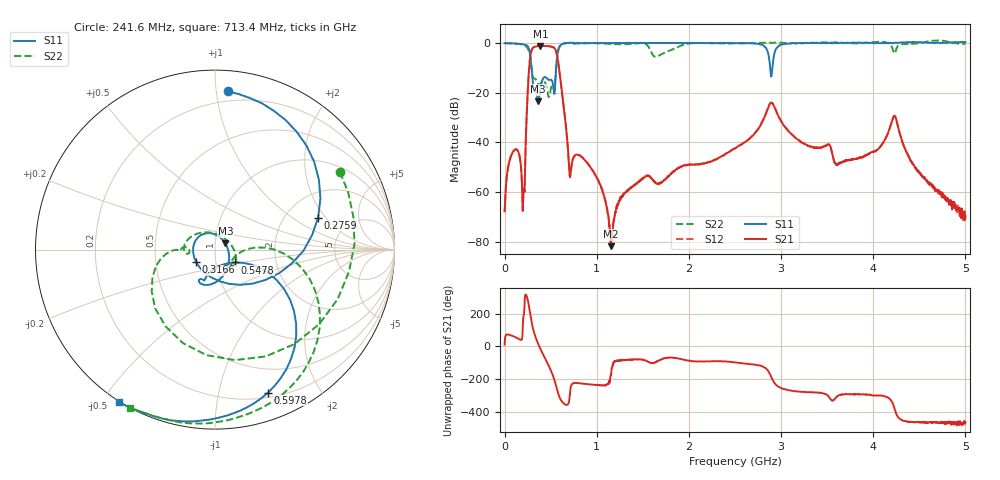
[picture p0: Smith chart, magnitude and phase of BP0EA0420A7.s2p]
!Agilent Technologies,E8358A,US41080443,A.07.50.56
!Agilent E8358A: A.07.50.56
!Date: Friday, November 10, 2017 09:12:03
!Correction: S11(Full 2 Port(1,2))
!S21(Full 2 Port(1,2))
!S12(Full 2 Port(1,2))
!S22(Full 2 Port(1,2))
!S2P File: Measurements: S11, S21, S12, S22:
# Hz S  dB  R 50
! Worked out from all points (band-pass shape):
!   1601 points, 1 MHz to 5 GHz, reference 50 ohm
!   highest |S21| = -1.22 dB at 388.4 MHz (marker M1); lowest = -81.7 dB at 1.157 GHz (marker M2)
!   |S21| within 3 dB of the highest: 285.1 MHz to 565.6 MHz (280.6 MHz wide, 66 % of centre)
!   lowest |S11| = -23.5 dB at 366.6 MHz (marker M3), VSWR 1.14, Z = 56 + j3.82 ohm
!   |S11| at or under -10 dB: 292.4 MHz to 559.8 MHz (267.3 MHz wide, 62.7 % of centre); 2.882 GHz to 2.905 GHz (23.26 MHz wide, 0.804 % of centre)
!   |S22| runs from -21.8 to 1.0 dB; largest |S21 - S12| = 0.005
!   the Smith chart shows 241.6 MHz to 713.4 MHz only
!   S11 on the Smith chart (normalised r, x): 241.6 MHz: 0.13, +1.08; 275.9 MHz: 2.99, +1.68; 316.6 MHz: 0.80, -0.11; 547.8 MHz: 1.23, -0.18; 597.8 MHz: 0.25, -1.41; 713.4 MHz: -0.00, -0.55
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1000000  -0.14 179.8  -67.48 10.5  -68.05 7.0  -0.14 179.8
1.041044e8  -0.25 156.7  -43.20 59.4  -43.09 59.6  -0.29 151.9
2.0096e8  -0.59 120.0  -64.21 159.2  -64.29 161.1  -0.78 99.7
2.415769e8  -1.07 85.4  -28.03 -55.3  -27.99 -55.3  -1.72 31.8
2.75945e8  -4.42 17.3  -6.55 -153.2  -6.51 -153.2  -5.19 -109.0
3.165619e8  -18.00 -146.0  -1.80 92.4  -1.76 92.4  -14.27 -178.2
3.665519e8  -23.49 30.5  -1.28 13.4  -1.24 13.5  -16.61 178.2
3.884225e8  -18.75 -50.7  -1.22 -14.3  -1.18 -14.3  -16.60 -171.9
4.634075e8  -14.38 -117.7  -1.30 -99.7  -1.27 -99.7  -19.39 116.0
5.477656e8  -17.64 -33.2  -2.39 142.7  -2.34 142.7  -16.40 -3.5
5.977556e8  -1.41 -69.6  -12.08 47.9  -12.04 48.0  -1.52 -54.0
7.133575e8  0.03 -122.3  -53.56 91.0  -53.49 90.8  0.01 -118.3
8.352081e8  -0.12 -140.4  -45.75 133.5  -45.68 133.5  -0.17 -136.4
1.157019e9  -0.05 -159.9  -81.67 -173.5  -79.56 -144.9  -0.42 -167.8
1.669416e9  -0.07 -172.7  -56.42 -88.1  -56.57 -88.5  -5.23 -135.2
2.5005e9  -0.15 170.8  -42.40 -98.3  -42.39 -98.3  -0.20 178.7
2.775445e9  -0.61 150.1  -33.20 -117.9  -33.20 -117.9  -0.03 171.7
2.891047e9  -13.27 12.7  -24.04 177.0  -24.05 177.0  0.02 175.3
3.006649e9  -0.67 -160.8  -31.75 103.6  -31.76 103.8  0.06 172.8
3.334708e9  -0.03 175.5  -41.84 78.8  -41.80 79.3  0.04 160.9
4.168916e9  0.00 159.9  -35.35 43.6  -35.36 44.2  -0.20 149.7
5e9  0.30 149.7  -69.51 -103.5  -70.74 -96.9  -0.46 154.6
